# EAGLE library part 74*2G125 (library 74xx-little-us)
Dual line drivers with 3-state outputs.
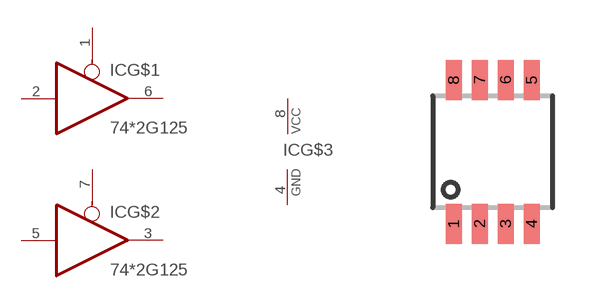
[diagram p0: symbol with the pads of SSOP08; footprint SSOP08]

Designator prefix IC; gates G$1=74125 G$2=74125 G$3=PWRN

## 74LVC2G125DCT  [SSOP08]
1  G$1:OE  in
2  G$1:I  in
3  G$2:O  hiz
4  G$3:GND  pwr
5  G$2:I  in
6  G$1:O  hiz
7  G$2:OE  in
8  G$3:VCC  pwr

## Footprint SSOP08 (pad centres in mm)
SMT SSOP 08
smd 0.4 x 1: 1 -0.975,-1.8; 2 -0.325,-1.8; 3 0.325,-1.8; 4 0.975,-1.8; 5 0.975,1.8; 6 0.325,1.8; 7 -0.325,1.8; 8 -0.975,1.8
